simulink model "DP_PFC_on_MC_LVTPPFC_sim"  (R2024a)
settings: Solver=odeN  StartTime=0.0  StopTime=1  FixedStep=Ts  MaxStep=10e-6  RelTol=1e-3  AbsTol=1e-4  EnableMultiTasking=on
PreLoadFcn:
  | TotemPole_PFCData;
StopFcn:
  | out.getSimulationMetadata.TimingInfo
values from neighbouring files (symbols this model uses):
  PWM = PWMType.Implementation    [TotemPole_PFCData.m]
  Ts = 5e-9    (= 5e-09)    [TotemPole_PFCData.m]
  Tsc_fast = 1e-5    (= 1e-05)    [TotemPole_PFCData.m]
  Tsc_slow = 0.01    [TotemPole_PFCData.m]
  Vrms = 23.0    (= 23)    [TotemPole_PFCData.m]
undefined symbols (not defined in the file or in its folder): AC, ADCs, ClosedLoop, Const, Detailed, Implementation, Inversion, Microchip, Noise, PI, Rnom, Simulation, ZenerResistiveLoad
libraries: fl_lib x23, nesl_utility x15, ee_lib x11, simulink x8, slctrl_fre x1, eeTotalHarmonicDistorsion x1
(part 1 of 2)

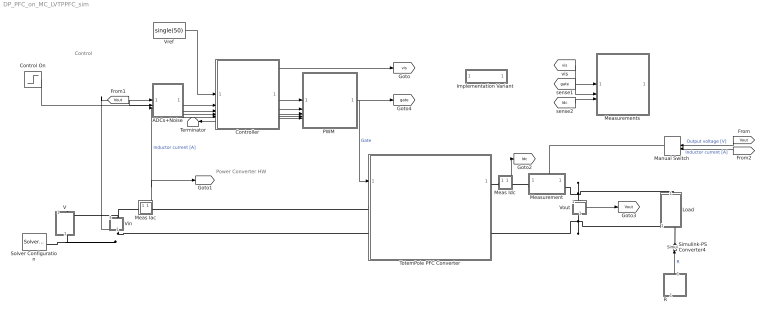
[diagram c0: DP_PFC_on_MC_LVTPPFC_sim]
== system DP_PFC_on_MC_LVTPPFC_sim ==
  note: Control
  note: Power Converter HW
  ADCs+Noise : Subsystem  Variant=on  VariantControl=ADCs+Noise
  Control On : Step  Time=0.12122  Before=1  After=0  SampleTime=0
  Controller : Subsystem  TreatAsAtomicUnit=on  ReferencedSubsystem=Control
  "Implementation Variant " : Subsystem  mask(Variant Selections){ImplVar=Simulation, VinVar=AC, ADCVar=Noise, ControlVar=Detailed, IControlVar=PI, PWMVar=Implementation, ConverterVar=Microchip, MeasureVar=ClosedLoop, LoadVar=ZenerResistiveLoad, RrefVar=Const}
      mask prompts: ImplVar "Implementation Variant"; VinVar "Vin Variant"; ADCVar "ADC Variant"; ControlVar "Control Variant"; IControlVar "IControl Variant"; PWMVar "PWM Variant"; ConverterVar "Converter Variant"; MeasureVar "Measurement Variant"; LoadVar "Load Variant"; RrefVar "Resistor Variant"
  Load : Subsystem  Variant=on  VariantControl=Subsystem
  Manual Switch : ManualSwitch  CurrentSetting=0
  Meas Iac : Subsystem
  Meas Idc : Subsystem
  Measurement : Subsystem  Variant=on  VariantControl=FrequencyResponse Measurement
  Measurements : Subsystem
  "PWM " : Subsystem  Variant=on  VariantControl=PWM+Inversion
  R : Subsystem  Variant=on  VariantControl=RLoadValue
  Simulink-PS Converter4 : nesl_utility/Simulink-PS Converter  PhysicalDomain=network_engine_domain  SubClassName=ps_input  LeftPortType=input  RightPortType=output  PseudoPeriodic=off  Frequencies=[]  NoiseDistribution=none  NoiseParameters=[]  Unit=Ohm  AffineConversion=off  FilteringAndDerivatives=provide  SimscapeFilterOrder=1  InputFilterTimeConstant=0.001  UdotUserProvided=0
  Solver Configuration : nesl_utility/Solver Configuration  PhysicalDomain=network_engine_domain  SubClassName=solver  LeftPortType=input  RightPortType=generic  Tones=[]  Harmonics=[]  SimulateNoise=off  Profile=off  UseLocalSampling=off  EnableSwitchedLinearOptims=on  FrequencyDomain=off  UseCCode=off  RelTol=0.001  AbsTol=1e-06  MinStep=1e-09  ToWorkspace=off  RevertToSquareIcSolve=off  NumHomotopyIterations=100  PhasorMode=off  PhasorModeNumHarmonics=1  ConsistencySolver=NEWTON_FTOL  IndexReductionMethod=DerivativeReplacement  DoDC=off  ResidualTolerance=1e-09  ConsistencyTolSource=GLOBAL  ConsistencyAbsTol=0.001  ConsistencyRelTol=0.001  ConsistencyTolFactor=0.001  UseLocalSolver=off  LocalSolverChoice=NE_PARTITIONING_ADVANCER  ResolveIndetEquations=off  FunctionEvalNumThread=1  LocalSolverSampleTime=Ts  DoFixedCost=off  MaxNonlinIter=3  MaxModeIter=2  ComputeImpulses=off  ImpulseIterations=2  LinearAlgebra=auto  LinearAlgebraNumThread=0  EquationFormulation=NE_TIME_EF  DelaysMemoryBudget=1024  AutomaticFiltering=on  FilteringTimeConstant=0.001  PartitionStorageMethod=AS_NEEDED  PartitionMemoryBudget=1024  PartitionMethod=FAST  MultibodyUseLocalSolver=off  MultibodyLocalSolverChoice=ODE1  MultibodyLocalSolverSampleTime=0.001
  Terminator : Terminator
  TotemPole PFC Converter : Subsystem  Variant=on  VariantControl=TotemPole PFC Converter
  V : Subsystem  Variant=on  VariantControl=Vin
  Vin : Subsystem
  Vout : Subsystem
  Vref : Constant  Value=single(50)  SampleTime=Tsc_slow
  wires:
  [vis] -> Measurements/1(In Bus Element)
  Vout/1(v) -> [Vout]
  Manual Switch/1 -> Measurement/1(y)
  [iL] -> Manual Switch/2  "Inductor current [A]"
  [Vout] -> Manual Switch/1  "Output voltage [V]"
  Meas Iac/1(i) -> [iL], ADCs+Noise/3(Iac)  "Inductor current [A]"
  "PWM "/1(Gate) -> [gate], TotemPole PFC Converter/1(G)  "Gate"
  [gate] -> Measurements/2(G)
  Meas Idc/1(i) -> [Idc]
  [Idc] -> Measurements/3(Idc)
  Vref/1 -> Controller/1
  Controller/1 -> [vis]
  Controller/2 -> "PWM "/1(DC)
  Controller/3 -> "PWM "/2(v_pos)
  Vin/1(v) -> ADCs+Noise/1(Vin)
  [Vout] -> ADCs+Noise/2(Vout)
  ADCs+Noise/1("Vin ") -> Controller/3
  ADCs+Noise/2("Vout ") -> Controller/4
  ADCs+Noise/3("Iac ") -> Controller/5
  R/1(Out1) -> Simulink-PS Converter4/1  "R"
  Controller/4 -> "PWM "/3(v_neg)
  Controller/5 -> "PWM "/4(v_zc)
  Control On/1 -> Controller/2
  Controller/6 -> "PWM "/5(PWM_Mode)
  Controller/7 -> Terminator/1
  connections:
  TotemPole PFC Converter/LConn1 -- Meas Iac/RConn1
  V/LConn1 -- Meas Iac/LConn1 -- Vin/LConn1
  Vin/RConn1 -- V/RConn1 -- Solver Configuration/RConn1 -- TotemPole PFC Converter/LConn2
  Measurement/LConn1 -- Meas Idc/RConn1
  TotemPole PFC Converter/RConn1 -- Meas Idc/LConn1
  Vout/RConn1 -- Load/LConn1 -- TotemPole PFC Converter/RConn2
  Vout/LConn1 -- Load/RConn1 -- Measurement/RConn1
  Simulink-PS Converter4/RConn1 -- Load/LConn2

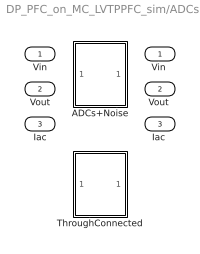
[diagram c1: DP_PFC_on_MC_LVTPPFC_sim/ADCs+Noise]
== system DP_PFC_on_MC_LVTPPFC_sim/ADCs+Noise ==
  Vin : Inport
  Vout : Inport  Port=2
  Iac : Inport  Port=3
  ADCs+Noise : Subsystem  VariantControl=ADC == ADCType.Noise
  ThroughConnected : Subsystem  VariantControl=ADC == ADCType.ThroughConnected
  "Vin " : Outport
  "Vout " : Outport  Port=2
  "Iac " : Outport  Port=3

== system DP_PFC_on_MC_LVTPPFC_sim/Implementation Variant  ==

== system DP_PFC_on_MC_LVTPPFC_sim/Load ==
  " ZenerD" : Subsystem  VariantControl=Load == LoadType.ZenerResistiveLoad
  VarR : Subsystem  VariantControl=Load ==LoadType.ResistiveLoad
  + : PMIOPort  Side=Right
  - : PMIOPort  Port=2  Side=Left
  R : PMIOPort  Port=3  Side=Left

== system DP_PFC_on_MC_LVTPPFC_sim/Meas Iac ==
  Current Sensor : fl_lib/Electrical/Electrical Sensors/Current Sensor
  PS-Simulink Converter1 : nesl_utility/PS-Simulink Converter  PhysicalDomain=network_engine_domain  SubClassName=ps_output  LeftPortType=input  RightPortType=output  PseudoPeriodic=off  Frequencies=[]  VectorFormat=1-D array  Unit=A  AffineConversion=off
  + : PMIOPort  Side=Left
  - : PMIOPort  Port=2  Side=Right
  i : Outport
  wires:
  PS-Simulink Converter1/1 -> i/1
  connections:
  +/RConn1 -- Current Sensor/LConn1
  Current Sensor/RConn1 -- PS-Simulink Converter1/LConn1
  Current Sensor/RConn2 -- -/RConn1

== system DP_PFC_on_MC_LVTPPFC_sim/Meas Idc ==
  Current Sensor : fl_lib/Electrical/Electrical Sensors/Current Sensor
  PS-Simulink Converter1 : nesl_utility/PS-Simulink Converter  PhysicalDomain=network_engine_domain  SubClassName=ps_output  LeftPortType=input  RightPortType=output  PseudoPeriodic=off  Frequencies=[]  VectorFormat=1-D array  Unit=A  AffineConversion=off
  - : PMIOPort  Side=Right
  + : PMIOPort  Port=2  Side=Left
  i : Outport
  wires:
  PS-Simulink Converter1/1 -> i/1
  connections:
  -/RConn1 -- Current Sensor/RConn2
  Current Sensor/RConn1 -- PS-Simulink Converter1/LConn1
  +/RConn1 -- Current Sensor/LConn1

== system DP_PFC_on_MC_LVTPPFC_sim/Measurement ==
  y : Inport
  ClsdLoop : Subsystem  VariantControl=Measure == MeasurementType.ClosedLoop
  FreqInj : Subsystem  VariantControl=Measure == MeasurementType.FrequencyInjection
  + : PMIOPort  Side=Left
  - : PMIOPort  Port=2  Side=Right

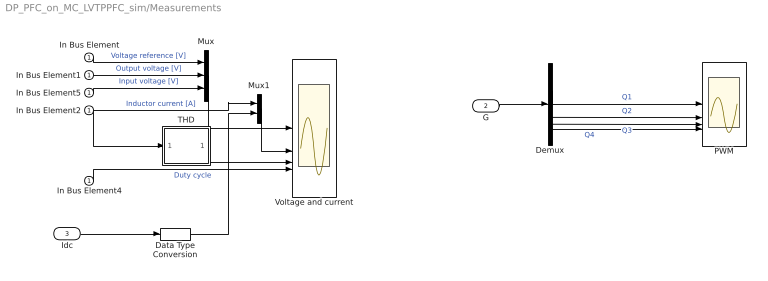
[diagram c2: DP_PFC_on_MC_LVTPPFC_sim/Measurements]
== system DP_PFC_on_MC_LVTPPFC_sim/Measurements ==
  In Bus Element{,1..2,4..5} (5 alike) : Inport
  G : Inport  Port=2
  Idc : Inport  Port=3  OutDataTypeStr=double
  Data Type Conversion : DataTypeConversion  OutDataTypeStr=single
  Demux : Demux
  Mux : Mux  Inputs=3
  Mux1 : Mux  Inputs=2
  PWM : Scope  NumInputPorts=4
  THD : Subsystem  Variant=on  VariantControl=THD
  Voltage and current : Scope  NumInputPorts=4
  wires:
  In Bus Element2/1 -> Mux1/1, THD/1(sig)  "Inductor current [A]"
  Mux/1 -> Voltage and current/1
  In Bus Element/1 -> Mux/1  "Voltage reference [V]"
  In Bus Element1/1 -> Mux/2  "Output voltage [V]"
  G/1 -> Demux/1
  Demux/1 -> PWM/1  "Q1"
  Demux/2 -> PWM/2  "Q2"
  Demux/3 -> PWM/3  "Q3"
  Demux/4 -> PWM/4  "Q4"
  In Bus Element4/1 -> Voltage and current/4  "Duty cycle"
  In Bus Element5/1 -> Mux/3  "Input voltage [V]"
  THD/1(THD) -> Voltage and current/3
  Mux1/1 -> Voltage and current/2
  Idc/1 -> Data Type Conversion/1
  Data Type Conversion/1 -> Mux1/2

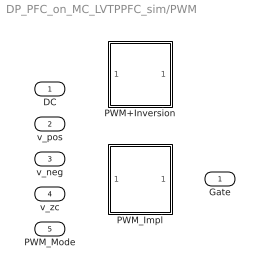
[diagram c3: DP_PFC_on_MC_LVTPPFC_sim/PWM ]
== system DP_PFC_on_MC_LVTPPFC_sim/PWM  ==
  DC : Inport
  v_pos : Inport  Port=2
  v_neg : Inport  Port=3
  v_zc : Inport  Port=4
  PWM_Mode : Inport  Port=5
  PWM+Inversion : Subsystem  VariantControl=PWM == PWMType.Concept
  PWM_Impl : Subsystem  VariantControl=PWM == PWMType.Implementation
  Gate : Outport

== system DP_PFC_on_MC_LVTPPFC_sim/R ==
  R_Const : Subsystem  VariantControl=Rref ==RrefType.Const
  R_Noisy : Subsystem  VariantControl=Rref ==RrefType.Noisy
  R_Stepped : Subsystem  VariantControl=Rref ==RrefType.Step
  Out1 : Outport

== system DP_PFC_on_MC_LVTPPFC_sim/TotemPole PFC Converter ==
  G : Inport
  "Ideal Switching, no thermal port" : Subsystem  VariantControl=Converter == ConverterType.Concept
  Microchip Ideal Switching : Subsystem  VariantControl=Converter == ConverterType.Microchip
  AC+ : PMIOPort  Side=Left
  AC- : PMIOPort  Port=2  Side=Left
  DC+ : PMIOPort  Port=3  Side=Right
  DC- : PMIOPort  Port=4  Side=Right

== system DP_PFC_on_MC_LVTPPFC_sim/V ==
  Vac : Subsystem  VariantControl=Vin == VinType.AC
  Vdc : Subsystem  VariantControl=Vin == VinType.DC
  + : PMIOPort  Side=Left
  - : PMIOPort  Port=2  Side=Right

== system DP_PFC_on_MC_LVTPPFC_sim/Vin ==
  PS-Simulink Converter : nesl_utility/PS-Simulink Converter  PhysicalDomain=network_engine_domain  SubClassName=ps_output  LeftPortType=input  RightPortType=output  PseudoPeriodic=off  Frequencies=[]  VectorFormat=1-D array  Unit=V  AffineConversion=off
  Voltage Sensor : fl_lib/Electrical/Electrical Sensors/Voltage Sensor
  + : PMIOPort  Side=Left
  - : PMIOPort  Port=2  Side=Right
  v : Outport
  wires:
  PS-Simulink Converter/1 -> v/1
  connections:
  Voltage Sensor/LConn1 -- +/RConn1
  Voltage Sensor/RConn2 -- -/RConn1
  PS-Simulink Converter/LConn1 -- Voltage Sensor/RConn1

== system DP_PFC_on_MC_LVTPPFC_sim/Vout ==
  PS-Simulink Converter : nesl_utility/PS-Simulink Converter  PhysicalDomain=network_engine_domain  SubClassName=ps_output  LeftPortType=input  RightPortType=output  PseudoPeriodic=off  Frequencies=[]  VectorFormat=1-D array  Unit=V  AffineConversion=off
  Voltage Sensor : fl_lib/Electrical/Electrical Sensors/Voltage Sensor
  + : PMIOPort  Side=Left
  - : PMIOPort  Port=2  Side=Right
  v : Outport
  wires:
  PS-Simulink Converter/1 -> v/1
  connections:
  PS-Simulink Converter/LConn1 -- Voltage Sensor/RConn1
  Voltage Sensor/RConn2 -- -/RConn1
  Voltage Sensor/LConn1 -- +/RConn1

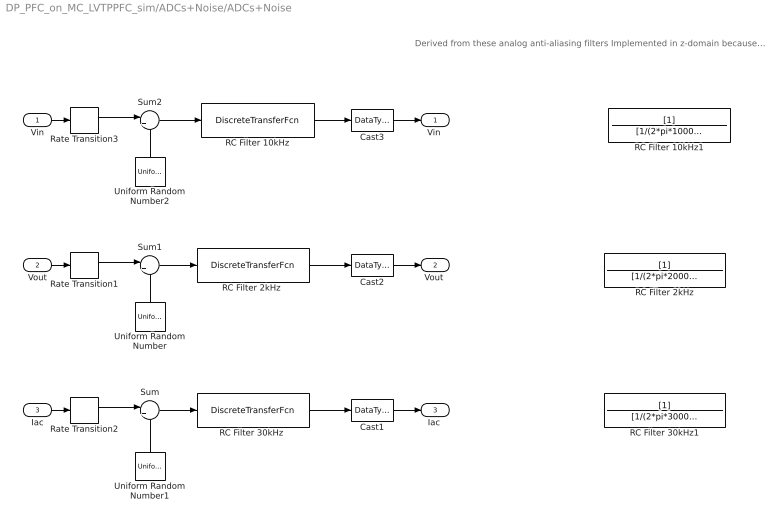
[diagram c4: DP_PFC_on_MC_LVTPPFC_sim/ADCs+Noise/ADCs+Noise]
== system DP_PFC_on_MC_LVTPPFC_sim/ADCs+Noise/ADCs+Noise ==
  note: Derived from these analog anti-aliasing filters Implemented in z-domain because noise added in z-domain
  Vin : Inport
  Vout : Inport  Port=2
  Iac : Inport  Port=3
  Cast1 : DataTypeConversion  OutDataTypeStr=single
  Cast2 : DataTypeConversion  OutDataTypeStr=single
  Cast3 : DataTypeConversion  OutDataTypeStr=single
  RC Filter 10kHz : DiscreteTransferFcn  Numerator=0.4665  Denominator=[1 -0.5335]
  RC Filter 10kHz1 : TransferFcn  Commented=on  Denominator=[1/(2*pi*10000) 1]
  RC Filter 2kHz : TransferFcn  Commented=on  Denominator=[1/(2*pi*2000) 1]
  "RC Filter 2kHz " : DiscreteTransferFcn  Numerator=0.06092  Denominator=[1 -0.9391]
  "RC Filter 30kHz " : DiscreteTransferFcn  Numerator=0.8482  Denominator=[1 -0.1518]
  RC Filter 30kHz1 : TransferFcn  Commented=on  Denominator=[1/(2*pi*30000) 1]
  Rate Transition1 : RateTransition  OutPortSampleTime=Tsc_fast
  Rate Transition2 : RateTransition  Deterministic=off  OutPortSampleTime=Tsc_fast
  Rate Transition3 : RateTransition  OutPortSampleTime=Tsc_fast
  Sum : Sum  Inputs=|++
  Sum1 : Sum  Inputs=|++
  Sum2 : Sum  Inputs=|++
  Uniform Random Number : UniformRandomNumber  Minimum=-0.01  Maximum=0.01  SampleTime=Tsc_fast
  Uniform Random Number1 : UniformRandomNumber  Minimum=-0.04  Maximum=0.04  Seed=1  SampleTime=Tsc_fast
  Uniform Random Number2 : UniformRandomNumber  Minimum=-0.01  Maximum=0.01  Seed=2  SampleTime=Tsc_fast
  "Vin " : Outport
  "Vout " : Outport  Port=2
  "Iac " : Outport  Port=3
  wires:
  Sum/1 -> "RC Filter 30kHz "/1
  Rate Transition2/1 -> Sum/1
  Rate Transition1/1 -> Sum1/1
  Uniform Random Number1/1 -> Sum/2
  Uniform Random Number/1 -> Sum1/2
  Sum1/1 -> "RC Filter 2kHz "/1
  Iac/1 -> Rate Transition2/1
  Cast2/1 -> "Vout "/1
  Vout/1 -> Rate Transition1/1
  Cast1/1 -> "Iac "/1
  Vin/1 -> Rate Transition3/1
  Cast3/1 -> "Vin "/1
  Sum2/1 -> RC Filter 10kHz/1
  Uniform Random Number2/1 -> Sum2/2
  Rate Transition3/1 -> Sum2/1
  RC Filter 10kHz/1 -> Cast3/1
  "RC Filter 2kHz "/1 -> Cast2/1
  "RC Filter 30kHz "/1 -> Cast1/1

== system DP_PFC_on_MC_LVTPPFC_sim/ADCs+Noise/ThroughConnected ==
  Vin : Inport
  Vout : Inport  Port=2
  Iac : Inport  Port=3
  "Vin " : Outport
  "Vout " : Outport  Port=2
  "Iac " : Outport  Port=3
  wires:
  Vin/1 -> "Vin "/1
  Iac/1 -> "Iac "/1
  Vout/1 -> "Vout "/1

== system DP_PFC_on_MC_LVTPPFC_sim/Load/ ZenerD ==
  Diode1 : ee_lib/Semiconductors & Converters/Diode  ModelType=ee.enum.diode.modelType.pwl  TableType=ee.enum.diode.tableType.IfMat  IfMat=[.07, .12, .19, 1.75, 4.24, 7.32, 11.2; .16, .3, .72, 2.14, 5.02, 8.35, 13.12] A  VfMat=[.9, 1.15, 1.25, 1.5, 1.75, 2.17, 2.6, 2.85; .58, .68, .75, 1.1, 1.38, 1.77, 2.27, 2.7] V  TjVec=[25, 125] degC  VfVec=[.5, .7, .9, 1.3, 1.7, 2.1, 2.5] V  IfVec=[.1, .2, .5, 1, 2, 4, 7, 10] A  IrMat=[1e-06, 2e-06, 5e-06, 1e-05, 2.5e-05, 5e-05, .0001; 2e-06, 5e-06, 1e-05, 4e-05, 8e-05, .0002, .0005] A  VrMat=[10, 100, 200, 250, 300, 325, 350; 10, 70, 160, 220, 270, 300, 320] V  VrVec=[10, 20, 40, 50, 70, 80, 100] V  IrVec=[1e-06, 2e-06, 5e-06, 1e-05, 2e-05, 5e-05, .0001] A  Vf=0.6 V  Ron=0.3 Ohm  Goff=1e-8 S  prmExp=ee.enum.diode.expParam.useTwo  I12=[.0137, .545] A  V12=[.6, .7] V  RS=0 Ohm  Tmeas=298.15 K  IS=1e-12 A  ec=1  I1=0.0137 A  V1=0.6 V  N_series=1  N_parallel=1  ZenerEnable=true  Rz=0.5 Ohm  BV=40 V  C_param=ee.enum.diode.capParam.fixed  CJ=0 pF  CJ0=5 pF  Vvec=[.1, 10, 100] V  Cvec=[3.5, 1, .4] pF  VJ=1 V  Mgrad=0.5  FC=0.5  Q_param=ee.enum.diode.recoveryParam.off  iRM=-7.15 A  iF=4 A  didt=-750 A/us  trr_factor=3  trr=115 ns  Qrr=150 nA*s  Vr=-600 V  Ls=150 nH  Erec=0.03 J  TT=50 ns  tau=100 ns  T_param=ee.enum.diode.temperatureParam.off  Tdevice=298.15 K  I1_T2=0.245 A  V1_T2=0.5 V  IS_T2=1.25e-7 A  Tmeas2=125 degC  XTI_param=ee.enum.diode.xtiParam.pn  XTI=3  EG_param=ee.enum.diode.egapParam.material_si  EG=1.11 eV  dBVdT=0 V/K  enable_faults=simscape.enum.onoff.off  fault_action=simscape.enum.assert.action.none  fault_types=ee.enum.diode.faults.open  tau_fault=1e-3 s  IfMat_faulted=[.07, .12, .19, 1.75, 4.24, 7.32, 11.2; .16, .3, .72, 2.14, 4.02, 6.35, 9.12] A  VfMat_faulted=[.9, 1.15, 1.25, 1.5, 1.75, 2.17, 2.6, 2.85; .58, .68, .75, 1.1, 1.38, 1.77, 2.27, 2.7] V  VfVec_faulted=[.5, .7, .9, 1.3, 1.7, 2.1, 2.5] V  IfVec_faulted=[.1, .2, .5, 1, 2, 4, 7, 10] A  IrMat_faulted=[1e-06, 2e-06, 5e-06, 1e-05, 2.5e-05, 5e-05, .0001; 2e-06, 5e-06, 1e-05, 4e-05, 8e-05, .0002, .0005] A  VrMat_faulted=[1, 10, 20, 25, 30, 32.5, 35; 1, 5, 10, 20, 25, 30, 32] V  VrVec_faulted=[1, 2, 4, 5, 7, 8, 10] V  IrVec_faulted=[1e-06, 2e-06, 5e-06, 1e-05, 2e-05, 5e-05, .0001] A  Ropen_faulted=1000 Ohm  Gshort_faulted=1000 1/Ohm  Vf_faulted=0.6 V  Ron_faulted=0.3 Ohm  Goff_faulted=1e-8 S  I12_faulted=[.0137, .545] A  V12_faulted=[.6, .7] V  IS_faulted=1e-12 A  ec_faulted=1  I1_faulted=0.0137 A  V1_faulted=0.6 V  RS_faulted=0 Ohm  Rz_faulted=0.3 Ohm  BV_faulted=inf V  Cscale_faulted=100  fault_trigger=ee.enum.faults.faultTrigger.temporal  t_fault=inf s  max_permissible_voltage=inf V  n_fail_on_voltage=1  max_permissible_current=inf A  t_fail_on_current=1 s  max_permissible_dVdt=inf V/s  enable_fault_input=simscape.enum.onoff.off  i_specify=off  i_priority=None  i=0 A  i_nominal_specify=off  i_nominal_value=1  i_nominal_unit=A  v_specify=off  v_priority=None  v=0 V  v_nominal_specify=off  v_nominal_value=1  v_nominal_unit=V  v_capacitor_specify=off  v_capacitor_priority=None  v_capacitor=0 V  v_capacitor_nominal_specify=off  v_capacitor_nominal_value=1  v_capacitor_nominal_unit=V  Qj_specify=off  Qj_priority=High  Qj=0 C  Qj_nominal_specify=off  Qj_nominal_value=1  Qj_nominal_unit=C  faulted_specify=off  faulted_priority=None  faulted=0  faulted_nominal_specify=off  faulted_nominal_value=1  faulted_nominal_unit=1  i_diode_specify=off  i_diode_priority=None  i_diode=0 A  i_diode_nominal_specify=off  i_diode_nominal_value=1  i_diode_nominal_unit=A  v_diode_specify=off  v_diode_priority=None  v_diode=0 V  v_diode_nominal_specify=off  v_diode_nominal_value=1  v_diode_nominal_unit=V  i_capacitor_specify=off  i_capacitor_priority=None  i_capacitor=0 A  i_capacitor_nominal_specify=off  i_capacitor_nominal_value=1  i_capacitor_nominal_unit=A  power_dissipated_specify=off  power_dissipated_priority=None  power_dissipated=0 W  power_dissipated_nominal_specify=off  power_dissipated_nominal_value=1  power_dissipated_nominal_unit=W  fidelity_level=ee.enum.diode.fidelity.includeChargeDyn  rec_loss_model=ee.enum.diode.reverseRecoveryModel.fixed  ErecVal=0 J  scaleWithIandV=true  ErecMat=zeros(2, 3) J  TjrecVec=[298.15, 398.15] K  IfrecVec=[.1, 1, 10] A  IrecVal=10 A  VrecVal=10 V  tFilter=1 / 1000 / 100 s  max_permissible_temperature=inf K  t_fail_on_temperature=1 s  thermal_network_parameterization=ee.enum.thermalNetworkTopology.junctionCase  Rth=[0, 10] K/W  Rth_Cauer=[1, 3, 10] K/W  Rth_Foster=[.08, .14, .22, .16] K/W  thermal_mass_parameterization=ee.enum.thermalNetwork.timeconstant  thermal_mass=[0, 1] J/K  thermal_mass_Cauer=[.1, .3, 1] J/K  thermal_mass_Foster=[.001, .005, .05, .5] J/K  thermal_time_constant=[0, 10] s  thermal_time_constant_Cauer=[1, 3, 10] s  thermal_time_constant_Foster=[7e-05, .0007, .01, .08] s  thermal_mass_initial_temperatures=[25, 25] degC  thermal_mass_initial_temperatures_Cauer=[25, 25, 25] degC  junction_thermal_mass=0.01 J/K  Tvec_initial_Foster=[25, 25, 25, 25] degC  no_thermal_network=0  junction_temperature_specify=off  junction_temperature_priority=None  junction_temperature=25 degC  junction_temperature_nominal_specify=off  junction_temperature_nominal_value=1  junction_temperature_nominal_unit=degC
  Variable Resistor1 : fl_lib/Electrical/Electrical Elements/Variable Resistor  Rmin=0 Ohm  thermalEnable=false  thermal_mass=1 J/K  i_specify=off  i_priority=None  i=0 A  i_nominal_specify=off  i_nominal_value=1  i_nominal_unit=A  v_specify=off  v_priority=None  v=0 V  v_nominal_specify=off  v_nominal_value=1  v_nominal_unit=V  T_specify=off  T_priority=None  T=300 K  T_nominal_specify=off  T_nominal_value=1  T_nominal_unit=K
  + : PMIOPort  Side=Right
  - : PMIOPort  Port=2  Side=Left
  R : PMIOPort  Port=3  Side=Left
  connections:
  Variable Resistor1/RConn1 -- -/RConn1
  Diode1/LConn1 -- Variable Resistor1/LConn2
  Variable Resistor1/LConn1 -- R/RConn1
  +/RConn1 -- Diode1/RConn1

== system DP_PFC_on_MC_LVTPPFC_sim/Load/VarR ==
  Variable Resistor : fl_lib/Electrical/Electrical Elements/Variable Resistor  Rmin=0 Ohm  thermalEnable=false  thermal_mass=1 J/K  i_specify=off  i_priority=None  i=0 A  i_nominal_specify=off  i_nominal_value=1  i_nominal_unit=A  v_specify=off  v_priority=None  v=0 V  v_nominal_specify=off  v_nominal_value=1  v_nominal_unit=V  T_specify=off  T_priority=None  T=300 K  T_nominal_specify=off  T_nominal_value=1  T_nominal_unit=K
  + : PMIOPort  Side=Right
  - : PMIOPort  Port=2  Side=Left
  R : PMIOPort  Port=3  Side=Left
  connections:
  Variable Resistor/LConn1 -- R/RConn1
  +/RConn1 -- Variable Resistor/LConn2
  -/RConn1 -- Variable Resistor/RConn1

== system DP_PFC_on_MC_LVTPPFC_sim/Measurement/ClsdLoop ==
  - : PMIOPort  Side=Right
  + : PMIOPort  Port=2  Side=Left
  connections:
  -/RConn1 -- +/RConn1

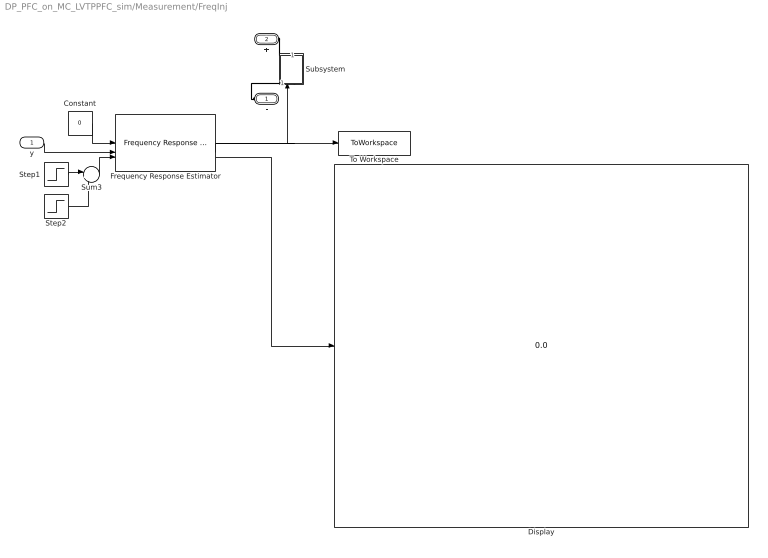
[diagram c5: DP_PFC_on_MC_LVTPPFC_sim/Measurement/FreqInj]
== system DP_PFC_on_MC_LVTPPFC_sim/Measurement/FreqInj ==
  y : Inport
  Constant : Constant  Value=0
  Display : Display
  Frequency Response Estimator : slctrl_fre/Frequency Response Estimator  DiscreteTs=Ts  OutputMode=perturbation only  BlockDataType=double  SineSource=Block parameters  Frequencies=logspace(1.5,4,100)  FreqUnits=Hz  Amplitudes=10  NumOfFreq=3  ExperimentMode=Sinestream  NumOfSetPeriod=4  NumOfEstPeriod=12  NumOfSlowestPeriod=3  NumOfPRBSPeriod=1  UseAutogenNumOfPRBSPeriod=off  PRBSSignalOrder=12  UseAutogenPRBSSignalOrder=off  EstimationMode=Online  UseBodePlot=on  BaselinePlant=[]  PlotRefreshFactor=100  UseExternalTs=off  BodePlotChoice=VariantBode  ExperimentChoice=VariantSS  OutputChoice=VariantDonly  CompiledTsChoice=InternalTs
  Step1 : Step  Time=3  SampleTime=0
  Step2 : Step  Time=50  After=-1  SampleTime=0
  Subsystem : Subsystem
  Sum3 : Sum  Inputs=|++
  To Workspace : ToWorkspace  VariableName=dataSS  SaveFormat=Timeseries  SampleTime=-1
  - : PMIOPort  Side=Right
  + : PMIOPort  Port=2  Side=Left
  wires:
  Frequency Response Estimator/1 -> Subsystem/1(V~)
  Step1/1 -> Sum3/1
  Step2/1 -> Sum3/2
  Sum3/1 -> Frequency Response Estimator/3
  Frequency Response Estimator/2 -> To Workspace/1
  Frequency Response Estimator/3 -> Display/1
  y/1 -> Frequency Response Estimator/2
  Constant/1 -> Frequency Response Estimator/1
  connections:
  -/RConn1 -- Subsystem/LConn1
  +/RConn1 -- Subsystem/RConn1

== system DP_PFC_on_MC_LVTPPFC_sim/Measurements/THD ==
  sig : Inport
  "THD " : Subsystem  VariantControl=THD == 1
  THD : Outport

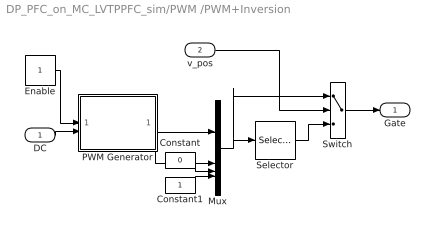
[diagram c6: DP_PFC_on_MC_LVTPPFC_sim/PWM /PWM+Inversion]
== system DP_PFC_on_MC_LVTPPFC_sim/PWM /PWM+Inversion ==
  DC : Inport
  v_pos : Inport  Port=2
  Constant : Constant  Value=0
  Constant1 : Constant
  Enable : Constant  SampleTime=Tsc_fast
  Mux : Mux
  PWM Generator : Subsystem  VariantControl=PWM == 2
  Selector : Selector  InputPortWidth=4  IndexOptions=Index vector (dialog)  Indices=[2 1 4 3]  OutputSizes=1
  Switch : Switch  Criteria=u2 ~= 0  Threshold=0.5
  Gate : Outport
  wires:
  Constant1/1 -> Mux/4
  Switch/1 -> Gate/1
  Mux/1 -> Selector/1, Switch/1
  PWM Generator/1(PWM_high) -> Mux/1
  Enable/1 -> PWM Generator/1(En)
  Constant/1 -> Mux/3
  PWM Generator/2(PWM_low) -> Mux/2
  Selector/1 -> Switch/3
  v_pos/1 -> Switch/2
  DC/1 -> PWM Generator/2(DC)

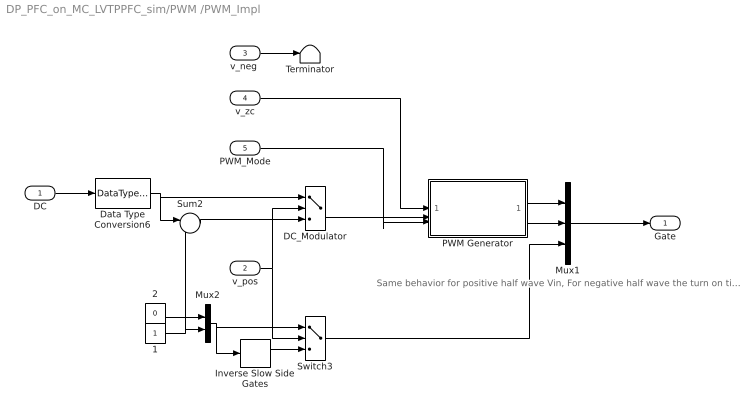
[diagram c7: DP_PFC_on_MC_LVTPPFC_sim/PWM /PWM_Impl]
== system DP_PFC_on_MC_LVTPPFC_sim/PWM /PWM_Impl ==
  note: Same behavior for positive half wave Vin, For negative half wave the turn on time is now still in miiddle and not at beginning and end
  DC : Inport
  v_pos : Inport  Port=2
  "v_neg " : Inport  Port=3
  v_zc : Inport  Port=4
  PWM_Mode : Inport  Port=5
  1 : Constant  OutDataTypeStr=double  SampleTime=Tsc_fast
  2 : Constant  Value=0  OutDataTypeStr=double  SampleTime=Tsc_fast
  DC_Modulator : Switch  Criteria=u2 ~= 0  Threshold=0.5  OutDataTypeStr=double  ZeroCross=off
  Data Type Conversion6 : DataTypeConversion  OutDataTypeStr=double
  Inverse Slow Side Gates : Selector  InputPortWidth=2  IndexOptions=Index vector (dialog)  Indices=[2 1]  OutputSizes=1
  Mux1 : Mux  Inputs=3
  Mux2 : Mux  Inputs=2
  PWM Generator : Subsystem  VariantControl=PWM == 2
  Sum2 : Sum  Inputs=|-+  OutDataTypeStr=double
  Switch3 : Switch  Criteria=u2 ~= 0  Threshold=0.5  OutDataTypeStr=double  ZeroCross=off
  Terminator : Terminator
  Gate : Outport
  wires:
  DC/1 -> Data Type Conversion6/1
  Mux2/1 -> Inverse Slow Side Gates/1, Switch3/1
  DC_Modulator/1 -> PWM Generator/2(DC)
  1/1 -> Mux2/2, Sum2/2
  Sum2/1 -> DC_Modulator/3
  2/1 -> Mux2/1
  Inverse Slow Side Gates/1 -> Switch3/3
  Switch3/1 -> Mux1/3
  PWM Generator/2(PWM_low) -> Mux1/2
  PWM Generator/1(PWM_high) -> Mux1/1
  Mux1/1 -> Gate/1
  Data Type Conversion6/1 -> Sum2/1, DC_Modulator/1
  v_zc/1 -> PWM Generator/1(v_zc)
  PWM_Mode/1 -> PWM Generator/3(PWM_Mode)
  v_pos/1 -> DC_Modulator/2, Switch3/2
  "v_neg "/1 -> Terminator/1

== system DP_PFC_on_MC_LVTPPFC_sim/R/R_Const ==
  Constant : Constant  Value=5
  Out1 : Outport
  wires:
  Constant/1 -> Out1/1

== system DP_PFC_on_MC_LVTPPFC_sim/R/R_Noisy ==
  RECORD : Scope
  Uniform Random Number : UniformRandomNumber  Minimum=Rnom*0.99  Maximum=Rnom *1.01  Seed=1  SampleTime=Tsc_fast
  Zero-Order Hold : ZeroOrderHold  SampleTime=Tsc_fast
  Out1 : Outport
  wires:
  Uniform Random Number/1 -> Zero-Order Hold/1, Out1/1
  Zero-Order Hold/1 -> RECORD/1

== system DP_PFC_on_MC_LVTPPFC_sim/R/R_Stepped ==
  Step : Step  Time=0.3  Before=120  After=120  SampleTime=0
  Out1 : Outport
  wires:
  Step/1 -> Out1/1

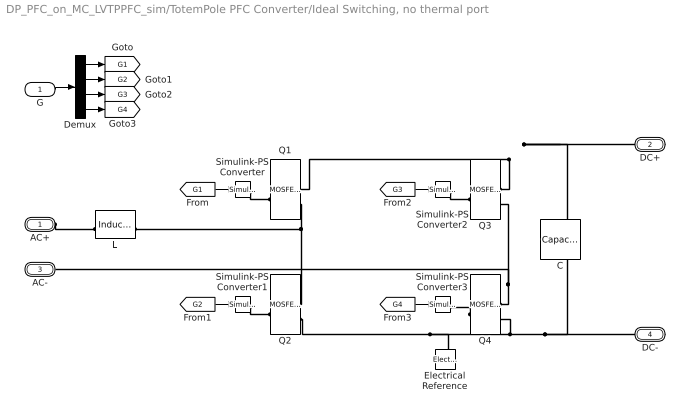
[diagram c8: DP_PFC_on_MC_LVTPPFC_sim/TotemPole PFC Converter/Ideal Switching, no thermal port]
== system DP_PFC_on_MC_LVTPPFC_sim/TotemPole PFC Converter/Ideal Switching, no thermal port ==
  G : Inport
  C : fl_lib/Electrical/Electrical Elements/Capacitor  c=8700 uF  r=0 Ohm  g=0 1/Ohm  i_specify=off  i_priority=None  i=0 A  i_nominal_specify=off  i_nominal_value=1  i_nominal_unit=A  v_specify=off  v_priority=High  v=0.1 V  v_nominal_specify=off  v_nominal_value=1  v_nominal_unit=V  vc_specify=off  vc_priority=High  vc=0 V  vc_nominal_specify=off  vc_nominal_value=1  vc_nominal_unit=V
  Demux : Demux
  Electrical Reference : fl_lib/Electrical/Electrical Elements/Electrical Reference
  L : fl_lib/Electrical/Electrical Elements/Inductor  l=266 uH  r=18 mOhm  g=0 1/Ohm  i_specify=off  i_priority=None  i=0 A  i_nominal_specify=off  i_nominal_value=1  i_nominal_unit=A  v_specify=off  v_priority=None  v=0 V  v_nominal_specify=off  v_nominal_value=1  v_nominal_unit=V  i_L_specify=off  i_L_priority=High  i_L=0 A  i_L_nominal_specify=off  i_L_nominal_value=1  i_L_nominal_unit=A
  Q1 : ee_lib/Semiconductors & Converters/MOSFET (Ideal, Switching)  port_option=ee.enum.controlport.ps  Rds=0.034 Ohm  Goff=1e-5 1/Ohm  Vth=0.5 V  diode_param=2  diode_Vf=3 V  diode_Ron=0.3 Ohm  diode_Goff=4e-5 1/Ohm  diode_C=50e-9 F  diode_iRM=-235 A  diode_iF=300 A  diode_idot=-50 A/us  diode_trr_param=1  diode_trr_factor=3  diode_trr=15 us  diode_Qrr=1500 s*uA  ids_specify=off  ids_priority=None  ids=0 A  ids_nominal_specify=off  ids_nominal_value=1  ids_nominal_unit=A  vds_specify=off  vds_priority=None  vds=0 V  vds_nominal_specify=off  vds_nominal_value=1  vds_nominal_unit=V  vgs_specify=off  vgs_priority=None  vgs=0 V  vgs_nominal_specify=off  vgs_nominal_value=1  vgs_nominal_unit=V  thermal_loss_option=ee.enum.converters.thermalLossOption.constantvalues  Von_data=[0, 1.8, 3.2, 6, 10, 16; 0, 2, 5.5, 9.5, 15, 25] V  Tj=[298.15, 448.15] K  Iout_data=[0, 20, 40, 60, 80, 100] A  Eon_data=[0, 55.04, 124.57, 235.53, 362.12; 0, 71.25, 161.25, 304.88, 468.75] * 1e-6 J  Eoff_data=[0, 18, 30, 56.1, 76.5; 0, 22.5, 37.5, 70.13, 95.63] * 1e-6 J  Eon_data_3D=[zeros(2, 5, 3)] J  Eoff_data_3D=[zeros(2, 5, 3)] J  Tj_loss=[298.15, 448.15] K  Iout_data_loss=[0, 10, 20, 30, 40] A  tabulateWithVds=false  Vds_loss=[0, 150, 300] V  Eon_scalar=22.86e-3 J  Eoff_scalar=17.14e-3 J  Voff=300 V  Iout_scalar=600 A  useCurrentFromPreviousCycle=false  useVoltageFromPreviousCycle=false  diodeModelType=ee.enum.converters.diodeModelType.pwl  diodeTableType=ee.enum.diode.tableType.IfMat  diode_ReverseIVType=ee.enum.diode.diodeReverseIV.constant  diode_IfMat=[.07, .12, .19, 1.75, 4.24, 7.32, 11.2; .16, .3, .72, 2.14, 4.02, 6.35, 9.12] A  diode_VfMat=[.9, 1.15, 1.25, 1.5, 1.75, 2.17, 2.6, 2.85; .58, .68, .75, 1.1, 1.38, 1.77, 2.27, 2.7] V  diode_TjVec=[25, 125] degC  diode_VfVec=[.5, .7, .9, 1.3, 1.7, 2.1, 2.5] V  diode_IfVec=[.1, .2, .5, 1, 2, 4, 7, 10] A  diode_IrMat=[1e-06, 2e-06, 5e-06, 1e-05, 2.5e-05, 5e-05, .0001; 2e-06, 5e-06, 1e-05, 4e-05, 8e-05, .0002, .0005] A  diode_VrMat=[10, 100, 200, 250, 300, 325, 350; 10, 70, 160, 220, 270, 300, 320] V  diode_VrVec=[10, 20, 40, 50, 70, 80, 100] V  diode_IrVec=[1e-06, 2e-06, 5e-06, 1e-05, 2e-05, 5e-05, .0001] A  diode_Vr=-600 V  diode_Ls=150 nH  diode_Erec=0.03 J  diode_rec_loss_model=ee.enum.diode.reverseRecoveryModel.fixed  diode_ErecVal=0 J  diode_scaleWithIandV=true  diode_ErecMat=zeros(2, 3) J  diode_TjrecVec=[298.15, 398.15] K  diode_IfrecVec=[.1, 1, 10] A  diode_IrecVal=10 A  diode_VrecVal=10 V  diode_tFilter=1 / 1000 / 100 s  thermal_network_parameterization=ee.enum.thermalNetworkTopology.external  Rth=[.03, .2] K/W  Rth_Cauer=[.03, .1, .2] K/W  Rth_Foster=[.03, .2] K/W  thermal_mass_parameterization=ee.enum.thermalNetwork.timeconstant  thermal_mass=[3, 25] J/K  thermal_mass_Cauer=[3, 10, 25] J/K  thermal_mass_Foster=[33, 50] J/K  thermal_time_constant=[.1, 5] s  thermal_time_constant_Cauer=[.1, 1, 5] s  thermal_time_constant_Foster=[1, 10] s  thermal_mass_initial_temperatures=[25, 25] degC  thermal_mass_initial_temperatures_Cauer=[25, 25, 25] degC  junction_thermal_mass=0.1 J/K  Tvec_initial_Foster=[25, 25, 25, 25] degC  no_thermal_network=0  junction_temperature_specify=off  junction_temperature_priority=None  junction_temperature=25 degC  junction_temperature_nominal_specify=off  junction_temperature_nominal_value=1  junction_temperature_nominal_unit=degC  Qj_specify=off  Qj_priority=None  Qj=0 W  Qj_nominal_specify=off  Qj_nominal_value=1  Qj_nominal_unit=W  accumulatedSwitchingLosses_specify=off  accumulatedSwitchingLosses_priority=None  accumulatedSwitchingLosses=0 J
  Q2 : ee_lib/Semiconductors & Converters/MOSFET (Ideal, Switching)  port_option=ee.enum.controlport.ps  Rds=0.034 Ohm  Goff=1e-5 1/Ohm  Vth=0.5 V  diode_param=2  diode_Vf=3 V  diode_Ron=0.3 Ohm  diode_Goff=4e-5 1/Ohm  diode_C=50e-9 F  diode_iRM=-235 A  diode_iF=300 A  diode_idot=-50 A/us  diode_trr_param=1  diode_trr_factor=3  diode_trr=15 us  diode_Qrr=1500 s*uA  ids_specify=off  ids_priority=None  ids=0 A  ids_nominal_specify=off  ids_nominal_value=1  ids_nominal_unit=A  vds_specify=off  vds_priority=None  vds=0 V  vds_nominal_specify=off  vds_nominal_value=1  vds_nominal_unit=V  vgs_specify=off  vgs_priority=None  vgs=0 V  vgs_nominal_specify=off  vgs_nominal_value=1  vgs_nominal_unit=V  thermal_loss_option=ee.enum.converters.thermalLossOption.constantvalues  Von_data=[0, 1.8, 3.2, 6, 10, 16; 0, 2, 5.5, 9.5, 15, 25] V  Tj=[298.15, 448.15] K  Iout_data=[0, 20, 40, 60, 80, 100] A  Eon_data=[0, 55.04, 124.57, 235.53, 362.12; 0, 71.25, 161.25, 304.88, 468.75] * 1e-6 J  Eoff_data=[0, 18, 30, 56.1, 76.5; 0, 22.5, 37.5, 70.13, 95.63] * 1e-6 J  Eon_data_3D=[zeros(2, 5, 3)] J  Eoff_data_3D=[zeros(2, 5, 3)] J  Tj_loss=[298.15, 448.15] K  Iout_data_loss=[0, 10, 20, 30, 40] A  tabulateWithVds=false  Vds_loss=[0, 150, 300] V  Eon_scalar=22.86e-3 J  Eoff_scalar=17.14e-3 J  Voff=300 V  Iout_scalar=600 A  useCurrentFromPreviousCycle=false  useVoltageFromPreviousCycle=false  diodeModelType=ee.enum.converters.diodeModelType.pwl  diodeTableType=ee.enum.diode.tableType.IfMat  diode_ReverseIVType=ee.enum.diode.diodeReverseIV.constant  diode_IfMat=[.07, .12, .19, 1.75, 4.24, 7.32, 11.2; .16, .3, .72, 2.14, 4.02, 6.35, 9.12] A  diode_VfMat=[.9, 1.15, 1.25, 1.5, 1.75, 2.17, 2.6, 2.85; .58, .68, .75, 1.1, 1.38, 1.77, 2.27, 2.7] V  diode_TjVec=[25, 125] degC  diode_VfVec=[.5, .7, .9, 1.3, 1.7, 2.1, 2.5] V  diode_IfVec=[.1, .2, .5, 1, 2, 4, 7, 10] A  diode_IrMat=[1e-06, 2e-06, 5e-06, 1e-05, 2.5e-05, 5e-05, .0001; 2e-06, 5e-06, 1e-05, 4e-05, 8e-05, .0002, .0005] A  diode_VrMat=[10, 100, 200, 250, 300, 325, 350; 10, 70, 160, 220, 270, 300, 320] V  diode_VrVec=[10, 20, 40, 50, 70, 80, 100] V  diode_IrVec=[1e-06, 2e-06, 5e-06, 1e-05, 2e-05, 5e-05, .0001] A  diode_Vr=-600 V  diode_Ls=150 nH  diode_Erec=0.03 J  diode_rec_loss_model=ee.enum.diode.reverseRecoveryModel.fixed  diode_ErecVal=0 J  diode_scaleWithIandV=true  diode_ErecMat=zeros(2, 3) J  diode_TjrecVec=[298.15, 398.15] K  diode_IfrecVec=[.1, 1, 10] A  diode_IrecVal=10 A  diode_VrecVal=10 V  diode_tFilter=1 / 1000 / 100 s  thermal_network_parameterization=ee.enum.thermalNetworkTopology.external  Rth=[.03, .2] K/W  Rth_Cauer=[.03, .1, .2] K/W  Rth_Foster=[.03, .2] K/W  thermal_mass_parameterization=ee.enum.thermalNetwork.timeconstant  thermal_mass=[3, 25] J/K  thermal_mass_Cauer=[3, 10, 25] J/K  thermal_mass_Foster=[33, 50] J/K  thermal_time_constant=[.1, 5] s  thermal_time_constant_Cauer=[.1, 1, 5] s  thermal_time_constant_Foster=[1, 10] s  thermal_mass_initial_temperatures=[25, 25] degC  thermal_mass_initial_temperatures_Cauer=[25, 25, 25] degC  junction_thermal_mass=0.1 J/K  Tvec_initial_Foster=[25, 25, 25, 25] degC  no_thermal_network=0  junction_temperature_specify=off  junction_temperature_priority=None  junction_temperature=25 degC  junction_temperature_nominal_specify=off  junction_temperature_nominal_value=1  junction_temperature_nominal_unit=degC  Qj_specify=off  Qj_priority=None  Qj=0 W  Qj_nominal_specify=off  Qj_nominal_value=1  Qj_nominal_unit=W  accumulatedSwitchingLosses_specify=off  accumulatedSwitchingLosses_priority=None  accumulatedSwitchingLosses=0 J
  Q3 : ee_lib/Semiconductors & Converters/MOSFET (Ideal, Switching)  port_option=ee.enum.controlport.ps  Rds=0.24 Ohm  Goff=1e-5 1/Ohm  Vth=0.5 V  diode_param=2  diode_Vf=0.6 V  diode_Ron=0.066 Ohm  diode_Goff=4e-5 1/Ohm  diode_C=50e-9 F  diode_iRM=-235 A  diode_iF=300 A  diode_idot=-50 A/us  diode_trr_param=1  diode_trr_factor=3  diode_trr=15 us  diode_Qrr=1500 s*uA  ids_specify=off  ids_priority=None  ids=0 A  ids_nominal_specify=off  ids_nominal_value=1  ids_nominal_unit=A  vds_specify=off  vds_priority=None  vds=0 V  vds_nominal_specify=off  vds_nominal_value=1  vds_nominal_unit=V  vgs_specify=off  vgs_priority=None  vgs=0 V  vgs_nominal_specify=off  vgs_nominal_value=1  vgs_nominal_unit=V  thermal_loss_option=ee.enum.converters.thermalLossOption.constantvalues  Von_data=[0, 1.8, 3.2, 6, 10, 16; 0, 2, 5.5, 9.5, 15, 25] V  Tj=[298.15, 448.15] K  Iout_data=[0, 20, 40, 60, 80, 100] A  Eon_data=[0, 55.04, 124.57, 235.53, 362.12; 0, 71.25, 161.25, 304.88, 468.75] * 1e-6 J  Eoff_data=[0, 18, 30, 56.1, 76.5; 0, 22.5, 37.5, 70.13, 95.63] * 1e-6 J  Eon_data_3D=[zeros(2, 5, 3)] J  Eoff_data_3D=[zeros(2, 5, 3)] J  Tj_loss=[298.15, 448.15] K  Iout_data_loss=[0, 10, 20, 30, 40] A  tabulateWithVds=false  Vds_loss=[0, 150, 300] V  Eon_scalar=22.86e-3 J  Eoff_scalar=17.14e-3 J  Voff=300 V  Iout_scalar=600 A  useCurrentFromPreviousCycle=false  useVoltageFromPreviousCycle=false  diodeModelType=ee.enum.converters.diodeModelType.pwl  diodeTableType=ee.enum.diode.tableType.IfMat  diode_ReverseIVType=ee.enum.diode.diodeReverseIV.constant  diode_IfMat=[.07, .12, .19, 1.75, 4.24, 7.32, 11.2; .16, .3, .72, 2.14, 4.02, 6.35, 9.12] A  diode_VfMat=[.9, 1.15, 1.25, 1.5, 1.75, 2.17, 2.6, 2.85; .58, .68, .75, 1.1, 1.38, 1.77, 2.27, 2.7] V  diode_TjVec=[25, 125] degC  diode_VfVec=[.5, .7, .9, 1.3, 1.7, 2.1, 2.5] V  diode_IfVec=[.1, .2, .5, 1, 2, 4, 7, 10] A  diode_IrMat=[1e-06, 2e-06, 5e-06, 1e-05, 2.5e-05, 5e-05, .0001; 2e-06, 5e-06, 1e-05, 4e-05, 8e-05, .0002, .0005] A  diode_VrMat=[10, 100, 200, 250, 300, 325, 350; 10, 70, 160, 220, 270, 300, 320] V  diode_VrVec=[10, 20, 40, 50, 70, 80, 100] V  diode_IrVec=[1e-06, 2e-06, 5e-06, 1e-05, 2e-05, 5e-05, .0001] A  diode_Vr=-600 V  diode_Ls=150 nH  diode_Erec=0.03 J  diode_rec_loss_model=ee.enum.diode.reverseRecoveryModel.fixed  diode_ErecVal=0 J  diode_scaleWithIandV=true  diode_ErecMat=zeros(2, 3) J  diode_TjrecVec=[298.15, 398.15] K  diode_IfrecVec=[.1, 1, 10] A  diode_IrecVal=10 A  diode_VrecVal=10 V  diode_tFilter=1 / 1000 / 100 s  thermal_network_parameterization=ee.enum.thermalNetworkTopology.external  Rth=[.03, .2] K/W  Rth_Cauer=[.03, .1, .2] K/W  Rth_Foster=[.03, .2] K/W  thermal_mass_parameterization=ee.enum.thermalNetwork.timeconstant  thermal_mass=[3, 25] J/K  thermal_mass_Cauer=[3, 10, 25] J/K  thermal_mass_Foster=[33, 50] J/K  thermal_time_constant=[.1, 5] s  thermal_time_constant_Cauer=[.1, 1, 5] s  thermal_time_constant_Foster=[1, 10] s  thermal_mass_initial_temperatures=[25, 25] degC  thermal_mass_initial_temperatures_Cauer=[25, 25, 25] degC  junction_thermal_mass=0.1 J/K  Tvec_initial_Foster=[25, 25, 25, 25] degC  no_thermal_network=0  junction_temperature_specify=off  junction_temperature_priority=None  junction_temperature=25 degC  junction_temperature_nominal_specify=off  junction_temperature_nominal_value=1  junction_temperature_nominal_unit=degC  Qj_specify=off  Qj_priority=None  Qj=0 W  Qj_nominal_specify=off  Qj_nominal_value=1  Qj_nominal_unit=W  accumulatedSwitchingLosses_specify=off  accumulatedSwitchingLosses_priority=None  accumulatedSwitchingLosses=0 J
  Q4 : ee_lib/Semiconductors & Converters/MOSFET (Ideal, Switching)  port_option=ee.enum.controlport.ps  Rds=0.24 Ohm  Goff=1e-5 1/Ohm  Vth=0.5 V  diode_param=2  diode_Vf=0.6 V  diode_Ron=0.066 Ohm  diode_Goff=4e-5 1/Ohm  diode_C=50e-9 F  diode_iRM=-235 A  diode_iF=300 A  diode_idot=-50 A/us  diode_trr_param=1  diode_trr_factor=3  diode_trr=15 us  diode_Qrr=1500 s*uA  ids_specify=off  ids_priority=None  ids=0 A  ids_nominal_specify=off  ids_nominal_value=1  ids_nominal_unit=A  vds_specify=off  vds_priority=None  vds=0 V  vds_nominal_specify=off  vds_nominal_value=1  vds_nominal_unit=V  vgs_specify=off  vgs_priority=None  vgs=0 V  vgs_nominal_specify=off  vgs_nominal_value=1  vgs_nominal_unit=V  thermal_loss_option=ee.enum.converters.thermalLossOption.constantvalues  Von_data=[0, 1.8, 3.2, 6, 10, 16; 0, 2, 5.5, 9.5, 15, 25] V  Tj=[298.15, 448.15] K  Iout_data=[0, 20, 40, 60, 80, 100] A  Eon_data=[0, 55.04, 124.57, 235.53, 362.12; 0, 71.25, 161.25, 304.88, 468.75] * 1e-6 J  Eoff_data=[0, 18, 30, 56.1, 76.5; 0, 22.5, 37.5, 70.13, 95.63] * 1e-6 J  Eon_data_3D=[zeros(2, 5, 3)] J  Eoff_data_3D=[zeros(2, 5, 3)] J  Tj_loss=[298.15, 448.15] K  Iout_data_loss=[0, 10, 20, 30, 40] A  tabulateWithVds=false  Vds_loss=[0, 150, 300] V  Eon_scalar=22.86e-3 J  Eoff_scalar=17.14e-3 J  Voff=300 V  Iout_scalar=600 A  useCurrentFromPreviousCycle=false  useVoltageFromPreviousCycle=false  diodeModelType=ee.enum.converters.diodeModelType.pwl  diodeTableType=ee.enum.diode.tableType.IfMat  diode_ReverseIVType=ee.enum.diode.diodeReverseIV.constant  diode_IfMat=[.07, .12, .19, 1.75, 4.24, 7.32, 11.2; .16, .3, .72, 2.14, 4.02, 6.35, 9.12] A  diode_VfMat=[.9, 1.15, 1.25, 1.5, 1.75, 2.17, 2.6, 2.85; .58, .68, .75, 1.1, 1.38, 1.77, 2.27, 2.7] V  diode_TjVec=[25, 125] degC  diode_VfVec=[.5, .7, .9, 1.3, 1.7, 2.1, 2.5] V  diode_IfVec=[.1, .2, .5, 1, 2, 4, 7, 10] A  diode_IrMat=[1e-06, 2e-06, 5e-06, 1e-05, 2.5e-05, 5e-05, .0001; 2e-06, 5e-06, 1e-05, 4e-05, 8e-05, .0002, .0005] A  diode_VrMat=[10, 100, 200, 250, 300, 325, 350; 10, 70, 160, 220, 270, 300, 320] V  diode_VrVec=[10, 20, 40, 50, 70, 80, 100] V  diode_IrVec=[1e-06, 2e-06, 5e-06, 1e-05, 2e-05, 5e-05, .0001] A  diode_Vr=-600 V  diode_Ls=150 nH  diode_Erec=0.03 J  diode_rec_loss_model=ee.enum.diode.reverseRecoveryModel.fixed  diode_ErecVal=0 J  diode_scaleWithIandV=true  diode_ErecMat=zeros(2, 3) J  diode_TjrecVec=[298.15, 398.15] K  diode_IfrecVec=[.1, 1, 10] A  diode_IrecVal=10 A  diode_VrecVal=10 V  diode_tFilter=1 / 1000 / 100 s  thermal_network_parameterization=ee.enum.thermalNetworkTopology.external  Rth=[.03, .2] K/W  Rth_Cauer=[.03, .1, .2] K/W  Rth_Foster=[.03, .2] K/W  thermal_mass_parameterization=ee.enum.thermalNetwork.timeconstant  thermal_mass=[3, 25] J/K  thermal_mass_Cauer=[3, 10, 25] J/K  thermal_mass_Foster=[33, 50] J/K  thermal_time_constant=[.1, 5] s  thermal_time_constant_Cauer=[.1, 1, 5] s  thermal_time_constant_Foster=[1, 10] s  thermal_mass_initial_temperatures=[25, 25] degC  thermal_mass_initial_temperatures_Cauer=[25, 25, 25] degC  junction_thermal_mass=0.1 J/K  Tvec_initial_Foster=[25, 25, 25, 25] degC  no_thermal_network=0  junction_temperature_specify=off  junction_temperature_priority=None  junction_temperature=25 degC  junction_temperature_nominal_specify=off  junction_temperature_nominal_value=1  junction_temperature_nominal_unit=degC  Qj_specify=off  Qj_priority=None  Qj=0 W  Qj_nominal_specify=off  Qj_nominal_value=1  Qj_nominal_unit=W  accumulatedSwitchingLosses_specify=off  accumulatedSwitchingLosses_priority=None  accumulatedSwitchingLosses=0 J
  Simulink-PS Converter{,1..3} (4 alike) : nesl_utility/Simulink-PS Converter  PhysicalDomain=network_engine_domain  SubClassName=ps_input  LeftPortType=input  RightPortType=output  PseudoPeriodic=off  Frequencies=[]  NoiseDistribution=none  NoiseParameters=[]  Unit=1  AffineConversion=off  FilteringAndDerivatives=provide  SimscapeFilterOrder=1  InputFilterTimeConstant=0.001  UdotUserProvided=0
  AC+ : PMIOPort  Side=Left
  DC+ : PMIOPort  Port=2  Side=Right
  AC- : PMIOPort  Port=3  Side=Left
  DC- : PMIOPort  Port=4  Side=Right
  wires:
  Demux/4 -> [G4]
  Demux/1 -> [G1]
  Demux/2 -> [G2]
  Demux/3 -> [G3]
  [G1] -> Simulink-PS Converter/1
  [G3] -> Simulink-PS Converter2/1
  [G2] -> Simulink-PS Converter1/1
  [G4] -> Simulink-PS Converter3/1
  G/1 -> Demux/1
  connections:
  Q4/RConn1 -- AC-/RConn1 -- Q3/RConn2
  Q2/RConn2 -- DC-/RConn1 -- C/RConn1 -- Q4/RConn2 -- Electrical Reference/LConn1
  L/RConn1 -- Q1/RConn2 -- Q2/RConn1
  Q3/RConn1 -- C/LConn1 -- DC+/RConn1 -- Q1/RConn1
  Simulink-PS Converter/RConn1 -- Q1/LConn1
  AC+/RConn1 -- L/LConn1
  Simulink-PS Converter1/RConn1 -- Q2/LConn1
  Simulink-PS Converter2/RConn1 -- Q3/LConn1
  Q4/LConn1 -- Simulink-PS Converter3/RConn1
